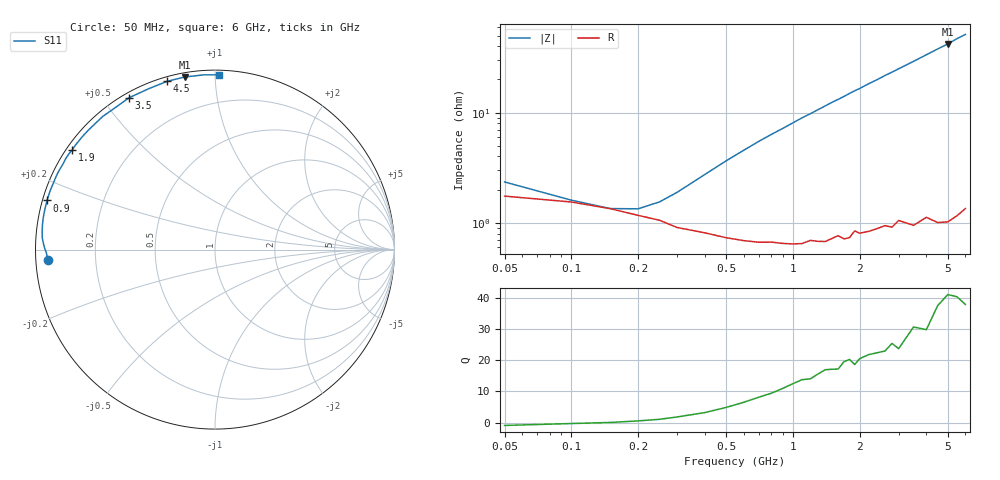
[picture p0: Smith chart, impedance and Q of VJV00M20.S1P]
! Infineon Technologies  Discrete & RF Semiconductors
! BB 914
! Si Tuning Diode in SOT23
! VR =
! S-Parameters:  July  1999
# GHz  S  MA  R  50
!  f  S11
! GHz  MAG  ANG
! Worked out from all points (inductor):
!   34 points, 50 MHz to 6 GHz, reference 50 ohm
!   read as one part to ground: L = 1.17 nH near 400 MHz
!   highest Q = 40.4 at 5 GHz (marker M1), where L = 1.34 nH
!   S11 on the Smith chart (normalised r, x): 50 MHz: 0.03, -0.03; 900 MHz: 0.01, +0.14; 1.9 GHz: 0.02, +0.32; 3.5 GHz: 0.02, +0.58; 4.5 GHz: 0.02, +0.76; 6 GHz: 0.03, +1.02
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0.05  0.9325 -176.4
0.1  0.94 -179.0
0.2  0.9543 178.5
0.3  0.9644 176.2
0.5  0.9713 171.8
0.6  0.973 169.7
0.8  0.974 165.6
0.9  0.9748 163.7
1.1  0.9752 159.7
1.2  0.9736 157.9
1.4  0.9746 154.1
1.5  0.9731 152.2
1.6  0.9718 150.5
1.7  0.9738 148.7
1.8  0.9734 146.8
1.9  0.9697 145.0
2  0.9714 143.4
2.2  0.9709 139.8
2.4  0.9698 136.6
2.6  0.9688 133.1
2.8  0.9704 130.1
3  0.9669 126.9
3.5  0.972 119.5
4  0.9695 112.4
4.5  0.9747 105.8
5  0.9763 100.0
5.5  0.9756 93.7
6  0.974 88.7
